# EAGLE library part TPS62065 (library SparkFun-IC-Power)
TPS62065 DC/DC step-Down regulator.
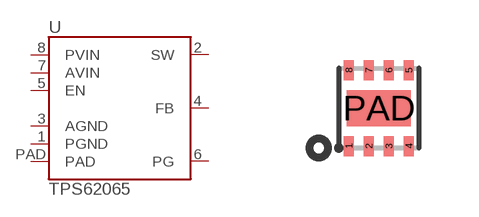
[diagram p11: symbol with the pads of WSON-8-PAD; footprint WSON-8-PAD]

Designator prefix U

## TPS62065 (PROD_ID: IC-12273)  [WSON-8-PAD]
1  PGND
2  SW
3  AGND
4  FB
5  EN
6  PG
7  AVIN
8  PVIN
PAD  PAD

## Footprint WSON-8-PAD (pad centres in mm)
smd 0.25 x 0.5: 1 -0.75,-0.95; 2 -0.25,-0.95; 3 0.25,-0.95; 4 0.75,-0.95; 5 0.75,0.95; 6 0.25,0.95; 7 -0.25,0.95; 8 -0.75,0.95
smd 1.6 x 0.9: PAD 0,0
